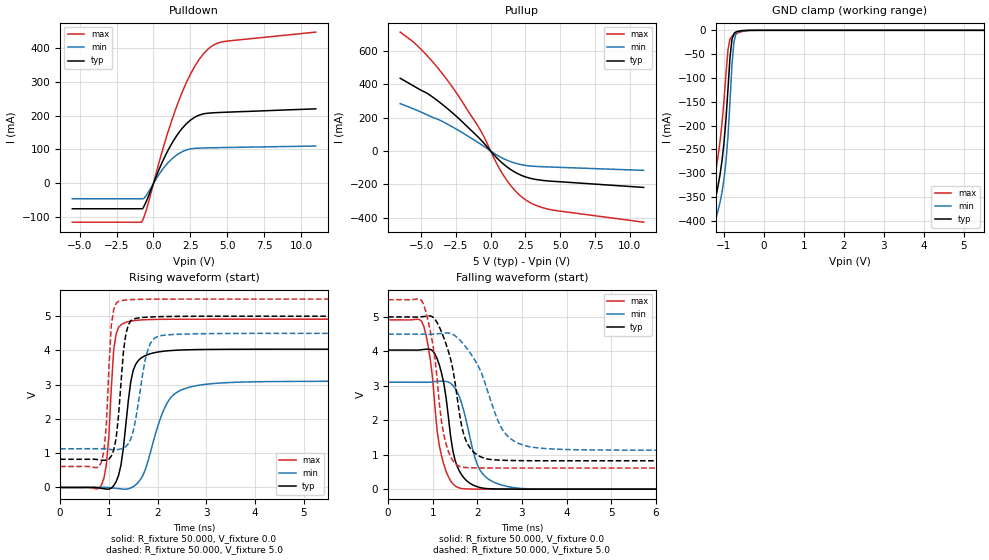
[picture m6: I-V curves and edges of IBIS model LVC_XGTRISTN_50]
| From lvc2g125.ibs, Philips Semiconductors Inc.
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|   Model LVC_XGTRISTN_50
[Model]   LVC_XGTRISTN_50
Model_type   3-state
Polarity   Non-Inverting
Enable   Active-Low
Vmeas =  2.5V
Cref  =  50.0pF
Rref  =  0.5k
Vref  =  0.0V
C_comp   3.70pF   2.73pF   4.99pF
[Model Spec]
| Note: The input and output voltage ratings may be exceeded if the input and
|   output current ratings are observed (please refer to the data sheet)
|   Subparameter   typ   min   max
| Timing Thresholds
Vmeas   2.5   2.25   2.75
|Ambient temperature:   25   85   -40
[Temperature Range]   50   105   -10
[Voltage Range]   5.0V   4.5V   5.5V
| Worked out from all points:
|   slope of the pulldown table from 0 to 0.75 V, typ, clamps not added: 9.74 ohm
|   slope of the pullup table from 0 to 0.75 V, typ, clamps not added: 11.5 ohm
|   GND clamp passes 1 mA (typ) near -0.56 V on its own axis
|   rising waveform, R_fixture 50.000, V_fixture 0.0: 20-80 % time 207ps typ, 433ps min, 127ps max; typ from 0 V to 4.04 V
|   rising waveform, R_fixture 50.000, V_fixture 5.0: 20-80 % time 153ps typ, 240ps min, 109ps max; typ from 0.823 V to 5 V
|   falling waveform, R_fixture 50.000, V_fixture 0.0: 20-80 % time 288ps typ, 383ps min, 269ps max; typ from 4.04 V to 0 V
|   falling waveform, R_fixture 50.000, V_fixture 5.0: 20-80 % time 371ps typ, 625ps min, 291ps max; typ from 5 V to 0.823 V
|Process Range   nominal   slow   fast
[Pulldown]
| voltage   I(typ)   I(min)   I(max)
-5.5V     -74.45mA   -44.94mA   -114mA
-800mV    -74.45mA   -44.94mA   -113.4mA
-700mV    -71.82mA   -44.94mA   -105mA
-450mV    -49.14mA   -32.48mA   -72.86mA
800mV     81.55mA    51.62mA    125.4mA
1.6V      142.4mA    84.6mA     230.2mA
2.2V      174.4mA    98.15mA    294.2mA
2.8V      195.1mA    103.4mA    345mA
3.7V      206.9mA    104.8mA    395.6mA
4.3V      208.6mA    105.3mA    412.3mA
4.9V      209.7mA    105.8mA    418.4mA
11V       219.7mA    110.2mA    445.6mA
[Pullup]
| voltage   I(typ)   I(min)   I(max)
-6.5V     436.3mA    284.4mA    713.8mA
-4.9V     360.6mA    230.1mA    601.6mA
-4.3V     331.8mA    207.1mA    547.7mA
-3.1V     254.6mA    161.4mA    424.1mA
-700mV    67mA       40.52mA    120.2mA
400mV     -36.99mA   -21.56mA   -69.19mA
1V        -83.39mA   -48.22mA   -155.6mA
1.6V      -119.2mA   -68.08mA   -222.6mA
2.4V      -151.7mA   -84.48mA   -285.7mA
3.2V      -169.4mA   -91.6mA    -323.6mA
4.4V      -180.8mA   -95.92mA   -352.6mA
11V       -217.8mA   -115.6mA   -426.5mA
[GND_clamp]
| voltage   I(typ)   I(min)   I(max)
-5.5V     -4.603A    -4.615A    -4.609A
-1.4V     -500.8mA   -542.2mA   -451.1mA
-1.35V    -454.6mA   -496.4mA   -404.6mA
-1.3V     -410.5mA   -452.8mA   -359.8mA
-1.25V    -373.2mA   -416.8mA   -320.9mA
-1.1V     -303.6mA   -361.8mA   -234.2mA
-1V       -236.4mA   -312.8mA   -148.1mA
-900mV    -123.4mA   -222.7mA   -41.02mA
-850mV    -57.76mA   -150.7mA   -18.63mA
-750mV    -6.642mA   -24.28mA   -9.684mA
-700mV    -3.294mA   -7.347mA   -7.431mA
5.5V      2.299nA    8.263nA    1.235nA
[Ramp]
| variable   typ   min   max
dV/dt_r   2.423V/207.198ps   1.862V/433.020ps   2.948V/127.419ps
dV/dt_f   2.506V/371.463ps   2.022V/625.054ps   2.932V/290.805ps
R_load = 50.000
[Rising Waveform]
R_fixture   = 50.000
V_fixture   = 0.0
V_fixture_min = 0.0
V_fixture_max = 0.0
| time   V(typ)   V(min)   V(max)
0s        299.3pV    3.653nV    23.62pV
850ps     -25.46mV   3.374mV    73.36mV
950ps     -48.3mV    2.481mV    678.4mV
1.1ns     51.15mV    -18.4mV    4.02V
1.35ns    1.847V     -49.76mV   4.819V
1.45ns    3.085V     -14.98mV   4.856V
1.6ns     3.697V     143.9mV    4.884V
2.2ns     3.988V     2.472V     4.91V
2.65ns    4.02V      2.925V     4.912V
9.75ns    4.038V     3.103V     4.913V
[Rising Waveform]
R_fixture   = 50.000
V_fixture   = 5.0
V_fixture_min = 4.5
V_fixture_max = 5.5
| time   V(typ)   V(min)   V(max)
0s        823mV      1.13V      612.8mV
850ps     796.9mV    1.131V     749.2mV
950ps     797.6mV    1.125V     1.846V
1.05ns    915.2mV    1.107V     4.725V
1.2ns     2.115V     1.111V     5.435V
1.3ns     3.969V     1.149V     5.465V
1.4ns     4.744V     1.275V     5.479V
1.8ns     4.973V     4.011V     5.496V
2.05ns    4.987V     4.424V     5.499V
9.75ns    5V         4.5V       5.5V
[Falling Waveform]
R_fixture   = 50.000
V_fixture   = 0.0
V_fixture_min = 0.0
V_fixture_max = 0.0
| time   V(typ)   V(min)   V(max)
0s        4.038V     3.104V     4.913V
800ps     4.056V     3.102V     4.727V
950ps     4.056V     3.108V     3.728V
1.15ns    3.599V     3.134V     1.257V
1.35ns    2.112V     3.109V     363.9mV
1.45ns    1.128V     3.016V     156.5mV
1.55ns    658.4mV    2.819V     57.51mV
2.05ns    51.25mV    577.1mV    1.098mV
2.6ns     3.43mV     101mV      -10.73uV
9.75ns    -564nV     -29.82uV   10.56pV
[Falling Waveform]
R_fixture   = 50.000
V_fixture   = 5.0
V_fixture_min = 4.5
V_fixture_max = 5.5
| time   V(typ)   V(min)   V(max)
0s        5V         4.5V       5.5V
800ps     5.012V     4.497V     5.349V
1.05ns    4.932V     4.504V     3.804V
1.25ns    4.391V     4.529V     1.572V
1.45ns    3.492V     4.493V     829mV
1.6ns     2.189V     4.34V      662mV
1.95ns    1.041V     3.734V     617.6mV
2.55ns    839.8mV    1.757V     613mV
3ns       827.5mV    1.29V      612.8mV
9.75ns    823mV      1.13V      612.8mV
